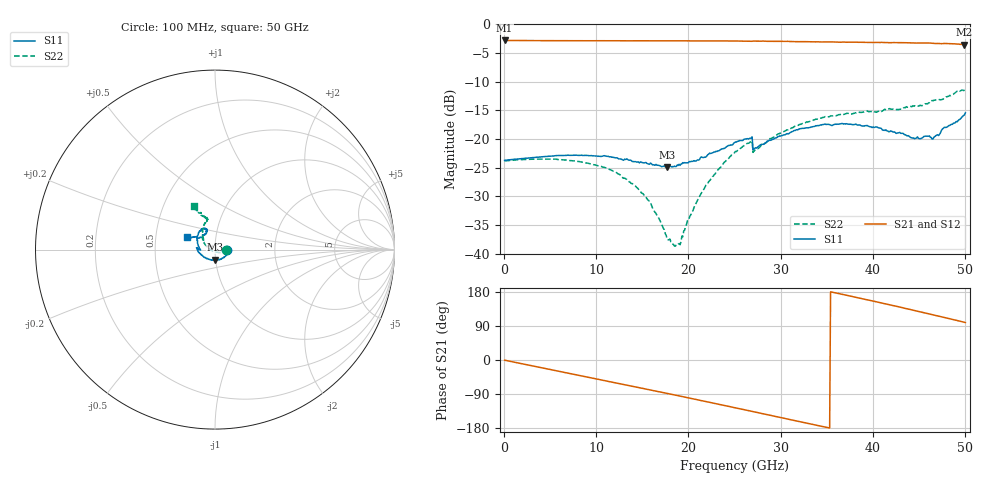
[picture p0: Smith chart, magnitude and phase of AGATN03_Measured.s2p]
! Filename4Jim: AG16_W2_AGATN03_D_0715_LRM_1BW_LRM.s2p
! Calibration: AG02 LRM + TRL
! Notes:
! Row:7, Col:15
! Probes: nan
! Prober: MPI TS150
! Date: 2023-09-21 10:44:34
! DC: None
# GHz S dB R 50
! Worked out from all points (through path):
!   500 points, 100 MHz to 50 GHz, reference 50 ohm
!   highest |S21| = -2.84 dB at 100 MHz (marker M1); lowest = -3.6 dB at 49.9 GHz (marker M2)
!   group delay of S21, straight-line fit = 14.4 ps
!   lowest |S11| = -24.9 dB at 17.7 GHz (marker M3), VSWR 1.12, Z = 49.9 - j5.68 ohm
!   |S11| at or under -10 dB: start of sweep to end of sweep
!   |S22| runs from -38.7 to -11.4 dB; largest |S21 - S12| = 0.0014
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0.1  -23.76 0.2  -2.84 -0.5  -2.84 -0.5  -23.88 0.3
4.2  -23.12 -1.6  -2.87 -20.8  -2.88 -20.8  -23.53 0.9
8.5  -22.89 -13.5  -2.89 -42.1  -2.89 -42.1  -24.07 -4.4
11.1  -22.99 -26.3  -2.89 -55.0  -2.89 -55.0  -25.11 -10.9
13.3  -23.51 -41.1  -2.90 -66.0  -2.90 -66.0  -27.03 -19.5
15.7  -24.40 -64.6  -2.89 -78.0  -2.89 -77.9  -30.72 -34.0
16.8  -24.63 -77.7  -2.89 -83.7  -2.89 -83.6  -33.85 -48.0
17.7  -24.92 -87.7  -2.91 -88.2  -2.91 -88.2  -37.52 -66.9
18.5  -24.77 -97.7  -2.90 -92.2  -2.90 -92.2  -38.69 -104.1
19  -24.43 -104.1  -2.89 -94.8  -2.90 -94.8  -38.26 -133.4
20  -24.19 -116.9  -2.91 -100.0  -2.91 -99.9  -34.25 -168.4
21.7  -23.22 -139.4  -2.91 -108.6  -2.91 -108.6  -28.74 168.1
25.1  -20.56 -172.4  -2.93 -126.2  -2.93 -126.2  -22.19 145.1
26.7  -19.89 174.5  -2.97 -134.5  -2.97 -134.5  -20.53 138.1
27.2  -21.64 178.5  -2.95 -137.3  -2.95 -137.2  -21.98 140.0
29.7  -19.61 159.3  -3.00 -150.2  -3.00 -150.2  -19.14 129.4
33.4  -17.91 137.0  -3.07 -169.7  -3.07 -169.6  -16.84 116.0
37.7  -17.50 118.8  -3.13 167.8  -3.13 167.8  -15.66 106.1
41.7  -18.76 113.3  -3.22 146.2  -3.22 146.2  -14.79 104.4
46.5  -19.98 136.3  -3.36 119.1  -3.36 119.2  -13.38 111.1
49.9  -15.83 156.0  -3.55 99.5  -3.56 99.5  -11.50 115.4
50  -15.46 156.3  -3.55 98.9  -3.55 99.0  -11.44 115.8
